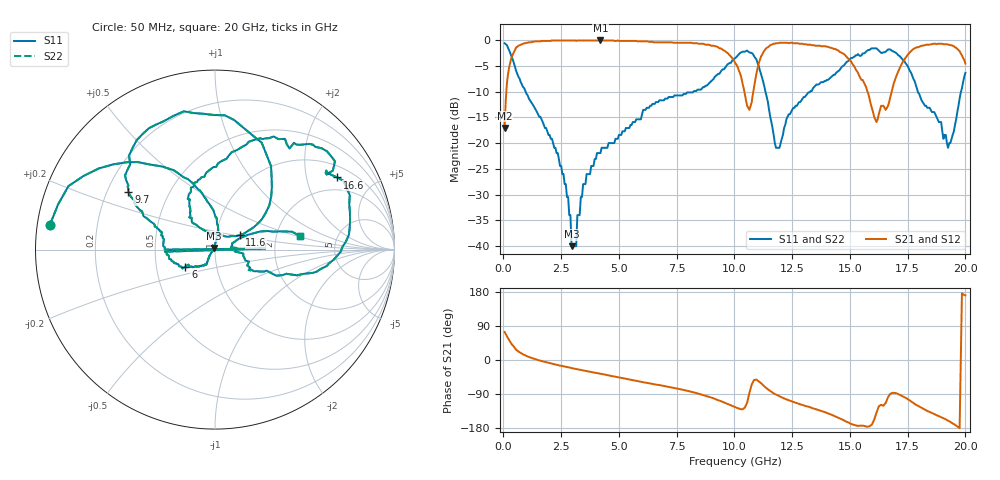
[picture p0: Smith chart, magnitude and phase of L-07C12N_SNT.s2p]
#	mhz	s	ma	r	50
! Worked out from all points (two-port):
!   400 points, 50 MHz to 20 GHz, reference 50 ohm
!   highest |S21| = -0.09 dB at 4.2 GHz (marker M1); lowest = -17.1 dB at 50 MHz (marker M2)
!   |S21| within 3 dB of the highest: 376.4 MHz to 9.823 GHz (9.446 GHz wide, 185 % of centre); 11.17 GHz to 14.82 GHz (3.654 GHz wide, 28.1 % of centre)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
!   lowest |S11| = -40.0 dB at 2.95 GHz (marker M3), VSWR 1.02, Z = 49.6 + j0.894 ohm
!   |S11| at or under -10 dB: 959.2 MHz to 8.231 GHz (7.272 GHz wide, 158 % of centre); 11.34 GHz to 13.28 GHz (1.94 GHz wide, 15.8 % of centre); 17.94 GHz to 19.81 GHz (1.872 GHz wide, 9.92 % of centre)
!   |S22| runs from -40.0 to -0.6 dB; largest |S21 - S12| = 0
!   S11 on the Smith chart (normalised r, x): 50 MHz: 0.04, +0.08; 6 GHz: 0.71, -0.14; 9.7 GHz: 0.29, +0.28; 11.6 GHz: 1.30, +0.22; 16.6 GHz: 1.42, +3.05; 20 GHz: 2.72, +0.54
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50  0.93 171.4  0.14 74.0  0.14 74.0  0.93 171.4
550  0.5 117.6  0.85 26.9  0.85 26.9  0.5 117.6
2950  0.01 115.6  0.99 -21.4  0.99 -21.4  0.01 115.6
3400  0.03 -137.1  0.99 -26.9  0.99 -26.9  0.03 -137.1
4200  0.08 -121.5  0.99 -36.4  0.99 -36.4  0.08 -121.5
6000  0.19 -150.2  0.97 -58.0  0.97 -58.0  0.19 -150.2
6700  0.25 -167.5  0.95 -65.7  0.95 -65.7  0.25 -167.5
7200  0.28 1.2  0.95 -71.4  0.95 -71.4  0.28 1.2
7250  0.28 180.0  0.95 -72.1  0.95 -72.1  0.28 180.0
9700  0.58 146.3  0.75 -115.9  0.75 -115.9  0.58 146.3
10050  0.67 134.8  0.59 -125.3  0.59 -125.3  0.67 134.8
10650  0.76 95.1  0.21 -86.5  0.21 -86.5  0.76 95.1
11600  0.16 30.6  0.9 -83.9  0.9 -83.9  0.16 30.6
13350  0.32 118.3  0.89 -126.5  0.89 -126.5  0.32 118.3
16600  0.79 30.6  0.22 -105.6  0.22 -105.6  0.79 30.6
16700  0.81 25.2  0.25 -93.7  0.25 -93.7  0.81 25.2
17750  0.42 -18.7  0.82 -113.3  0.82 -113.3  0.42 -18.7
19600  0.17 24.4  0.84 -173.2  0.84 -173.2  0.17 24.4
19750  0.27 21.9  0.78 -179.9  0.78 -179.9  0.27 21.9
19800  0.31 19.5  0.74 -2.1  0.74 -2.1  0.31 19.5
19850  0.34 17.1  0.71 175.6  0.71 175.6  0.34 17.1
20000  0.48 9.1  0.59 170.7  0.59 170.7  0.48 9.1
